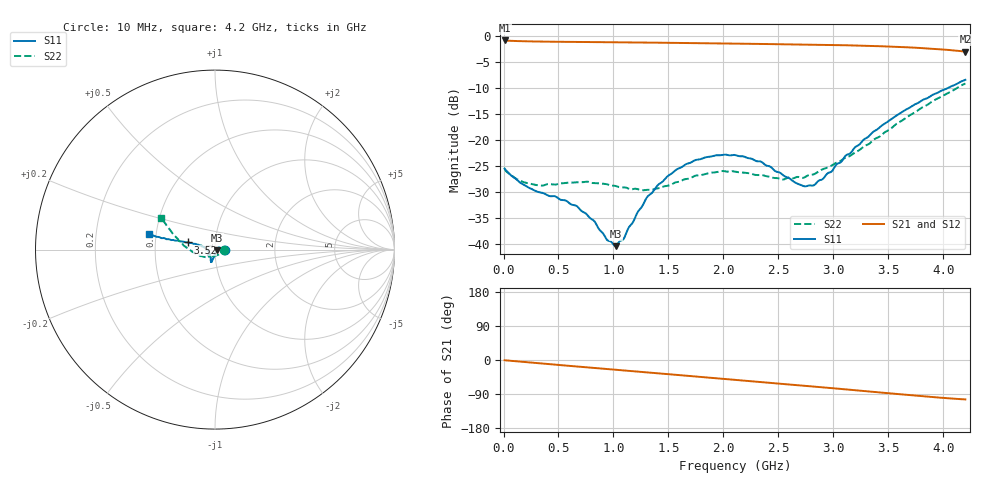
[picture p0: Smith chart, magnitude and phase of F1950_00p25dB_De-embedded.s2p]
! Integrated Device Technology
! Corporate Headquarters
! 6024 Silver Creek Valley Road
! San Jose, CA 95138  USA
! Phone:  1-408-284-8200
! Toll Free:  1-800-223-1366
! Webpage:  http://www.idt.com/
! Timing and RF Division
! 515 Groton Road, Suite 102
! Westford, MA 01886-6024
! Device:  F1950
! Description: 7-bit 0.25 dB Digital Step Attenuator
! Frequency:  150.0 -  4000.00 MHz
! Package:  4x4 mm Thin QFN Plastic Package: 24 pin
! Ports:  2 RF, 12 DC
!  Pin  1  = D0
!  Pin  2  = VDD
!  Pin  3  = Vmode
!  Pin  4  = GND
!  Pin  5  = RF1  =  Port 1
!  Pin  6  = GND
!  Pin  7  = GND
!  Pin  8  = GND
!  Pin  9  = GND
!  Pin 10  = GND
!  Pin 11  = GND
!  Pin 12  = GND
!  Pin 13  = GND
!  Pin 14  = RF2  =  Port 2
!  Pin 15  = GND
!  Pin 16  = LE
!  Pin 17  = CLK
!  Pin 18  = DATE
!  Pin 19  = D6
!  Pin 20  = D5
!  Pin 21  = D4
!  Pin 22  = D3
!  Pin 23  = D2
!  Pin 24  = D1
! State:  1
! Atten State:  0.25 dB
! Voltage:  +5.00 Volts
! Current:  Not Measured mA
! Data:  The device was measured on a the F195X evaluation board which has
!  individual transmission lines to the RF pins.  Data was collected
!  using a calibrated network analyzer.  The evaluation board was
!  de-embedded using a TRL calibration technique.
!  The reference plane is the edge of the package pin.
! Misc:  Board 2019
!  Action Tracker AT0250
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# GHz S dB R 50
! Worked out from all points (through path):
!   420 points, 10 MHz to 4.2 GHz, reference 50 ohm
!   highest |S21| = -0.90 dB at 10 MHz (marker M1); lowest = -3.0 dB at 4.2 GHz (marker M2)
!   group delay of S21, straight-line fit = 69 ps
!   lowest |S11| = -40.4 dB at 1.02 GHz (marker M3), VSWR 1.02, Z = 50.9 - j0.437 ohm
!   |S11| at or under -10 dB: start of sweep to 4.043 GHz
!   |S22| runs from -29.6 to -9.2 dB; largest |S21 - S12| = 0.0011
!   S11 on the Smith chart (normalised r, x): 10 MHz: 1.11, -0.01; 3.52 GHz: 0.73, +0.06; 4.2 GHz: 0.46, +0.09
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0.01  -25.47 -3.2  -0.90 -0.7  -0.90 -0.7  -25.55 -4.6
0.13  -27.79 -5.7  -1.02 -4.0  -1.02 -4.0  -27.60 -5.8
0.29  -29.77 8.0  -1.10 -8.0  -1.10 -8.0  -28.61 -0.6
0.57  -31.66 26.8  -1.17 -14.8  -1.17 -14.8  -28.23 2.2
0.71  -33.64 28.5  -1.19 -18.2  -1.19 -18.2  -28.11 -4.6
0.82  -35.45 23.6  -1.21 -20.9  -1.21 -20.9  -28.27 -10.7
0.94  -39.15 4.6  -1.24 -23.8  -1.24 -23.8  -28.48 -21.1
1.02  -40.37 -26.6  -1.25 -25.7  -1.25 -25.7  -28.83 -30.0
1.09  -39.04 -57.4  -1.27 -27.4  -1.26 -27.4  -29.09 -38.8
1.3  -31.13 -93.2  -1.30 -32.6  -1.30 -32.6  -29.58 -70.2
1.41  -28.52 -97.9  -1.33 -35.3  -1.33 -35.3  -29.26 -87.2
1.57  -25.71 -102.2  -1.37 -39.2  -1.37 -39.2  -28.11 -108.9
1.74  -23.89 -104.6  -1.41 -43.3  -1.41 -43.4  -26.88 -125.1
2.11  -22.90 -108.0  -1.51 -52.4  -1.51 -52.4  -26.09 -141.8
2.34  -24.15 -113.2  -1.57 -58.0  -1.57 -58.1  -26.71 -141.3
2.54  -26.71 -121.9  -1.62 -62.9  -1.62 -63.0  -27.59 -134.9
2.72  -28.79 -146.2  -1.67 -67.5  -1.67 -67.5  -27.27 -128.3
2.81  -28.75 -161.5  -1.70 -69.7  -1.70 -69.8  -26.64 -127.8
3.15  -22.61 165.5  -1.84 -78.5  -1.83 -78.6  -23.06 -144.9
3.51  -16.24 165.1  -2.07 -87.9  -2.06 -88.0  -18.01 -174.2
3.52  -16.09 165.4  -2.07 -88.2  -2.07 -88.2  -17.86 -175.1
4.2  -8.45 166.9  -3.03 -104.1  -3.02 -104.1  -9.17 149.2
